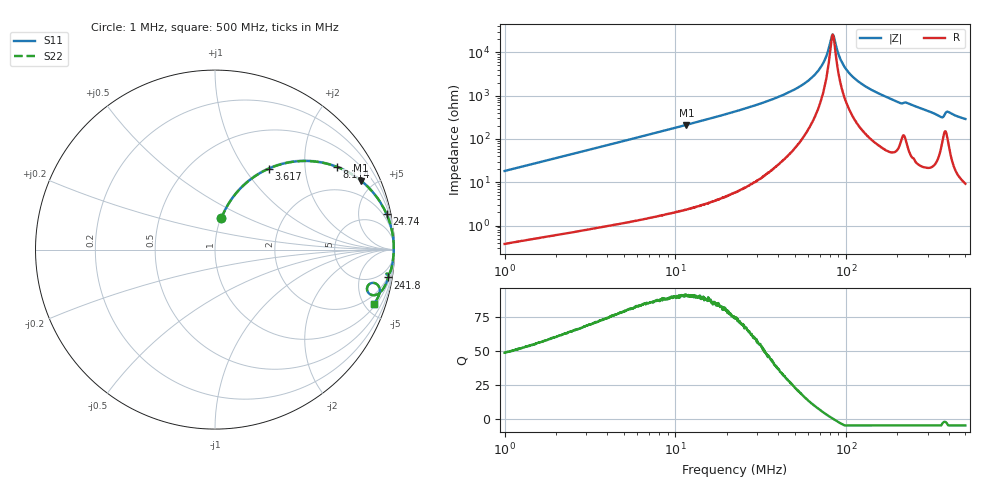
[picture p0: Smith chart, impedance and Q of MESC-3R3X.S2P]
!s-Parameter Generated by FASTRON Sdn. Bhd.
!FASTRON P/N : MESC-3R3X
!Keysight Technologies,E4991B,MY54100416,A.01.15
!Date: Mon Mar 16 10:48:25 2026
!Version  : Rev00 Mon Mar 16 10:48:25 2026
!Data & Calibration Information:
!PortZ  Port1:50+j0  Port2:50+j0
!When reading, reference impedance value at option line is always used.
!Remarks : This data is being provided solely for informational purposes.
!Freq	S11	S21	S12	S22
# Hz S dB R 50
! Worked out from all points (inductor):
!   1601 points, 1 MHz to 500 MHz, reference 50 ohm
!   read as one part in series: L = 2.89 uH near 1.032 MHz
!   highest Q = 90.8 at 11.6 MHz (marker M1), where L = 2.9 uH
!   self-resonance near 83.43 MHz
!   S11 on the Smith chart (normalised r, x): 1 MHz: 1.01, +0.36; 3.617 MHz: 1.02, +1.30; 8.114 MHz: 1.03, +2.93; 24.74 MHz: 1.14, +9.68; 241.8 MHz: 2, -12; 500 MHz: 1.18, -5.79
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1000000  -14.97 78.5  -0.17 -10.3  -0.17 -10.3  -14.97 78.5
2820919  -6.92 62.4  -1.05 -26.8  -1.05 -26.8  -6.92 62.4
3617008  -5.31 56.4  -1.59 -32.8  -1.59 -32.8  -5.31 56.4
7957584  -1.76 34.6  -4.91 -54.7  -4.91 -54.7  -1.76 34.6
8113636  -1.71 34.1  -5.03 -55.2  -5.03 -55.2  -1.71 34.1
1.159862e7  -0.91 25.2  -7.41 -64.2  -7.41 -64.2  -0.91 25.2
2.236068e7  -0.25 13.1  -12.92 -76.2  -12.92 -76.2  -0.25 13.1
2.473679e7  -0.21 11.6  -13.91 -77.5  -13.91 -77.5  -0.21 11.6
4.446912e7  -0.06 5.1  -20.98 -83.0  -20.98 -83.0  -0.06 5.1
6.307767e7  -0.04 2.2  -28.39 -82.7  -28.39 -82.7  -0.04 2.2
7.339442e7  -0.03 1.0  -35.03 -77.2  -35.03 -77.2  -0.03 1.0
7.719553e7  -0.03 0.6  -38.98 -69.8  -38.98 -69.8  -0.03 0.6
8.182669e7  -0.03 0.2  -46.46 -36.1  -46.46 -36.1  -0.03 0.2
8.375604e7  -0.03 -0.0  -48.15 4.3  -48.15 4.3  -0.03 -0.0
9.374216e7  -0.04 -0.9  -36.02 74.1  -36.02 74.1  -0.04 -0.9
1.057371e8  -0.04 -1.8  -29.95 80.3  -29.95 80.3  -0.04 -1.8
1.294029e8  -0.06 -3.4  -24.42 81.9  -24.42 81.9  -0.06 -3.4
1.77937e8  -0.11 -6.4  -19.03 80.3  -19.03 80.3  -0.11 -6.4
2.418399e8  -0.20 -9.1  -15.95 77.2  -15.95 77.2  -0.20 -9.1
3.538668e8  -0.70 -16.0  -11.12 66.0  -11.12 66.0  -0.70 -16.0
3.929931e8  -0.66 -12.2  -13.25 64.2  -13.25 64.2  -0.66 -12.2
5e8  -0.57 -18.9  -9.81 69.3  -9.81 69.3  -0.57 -18.9
